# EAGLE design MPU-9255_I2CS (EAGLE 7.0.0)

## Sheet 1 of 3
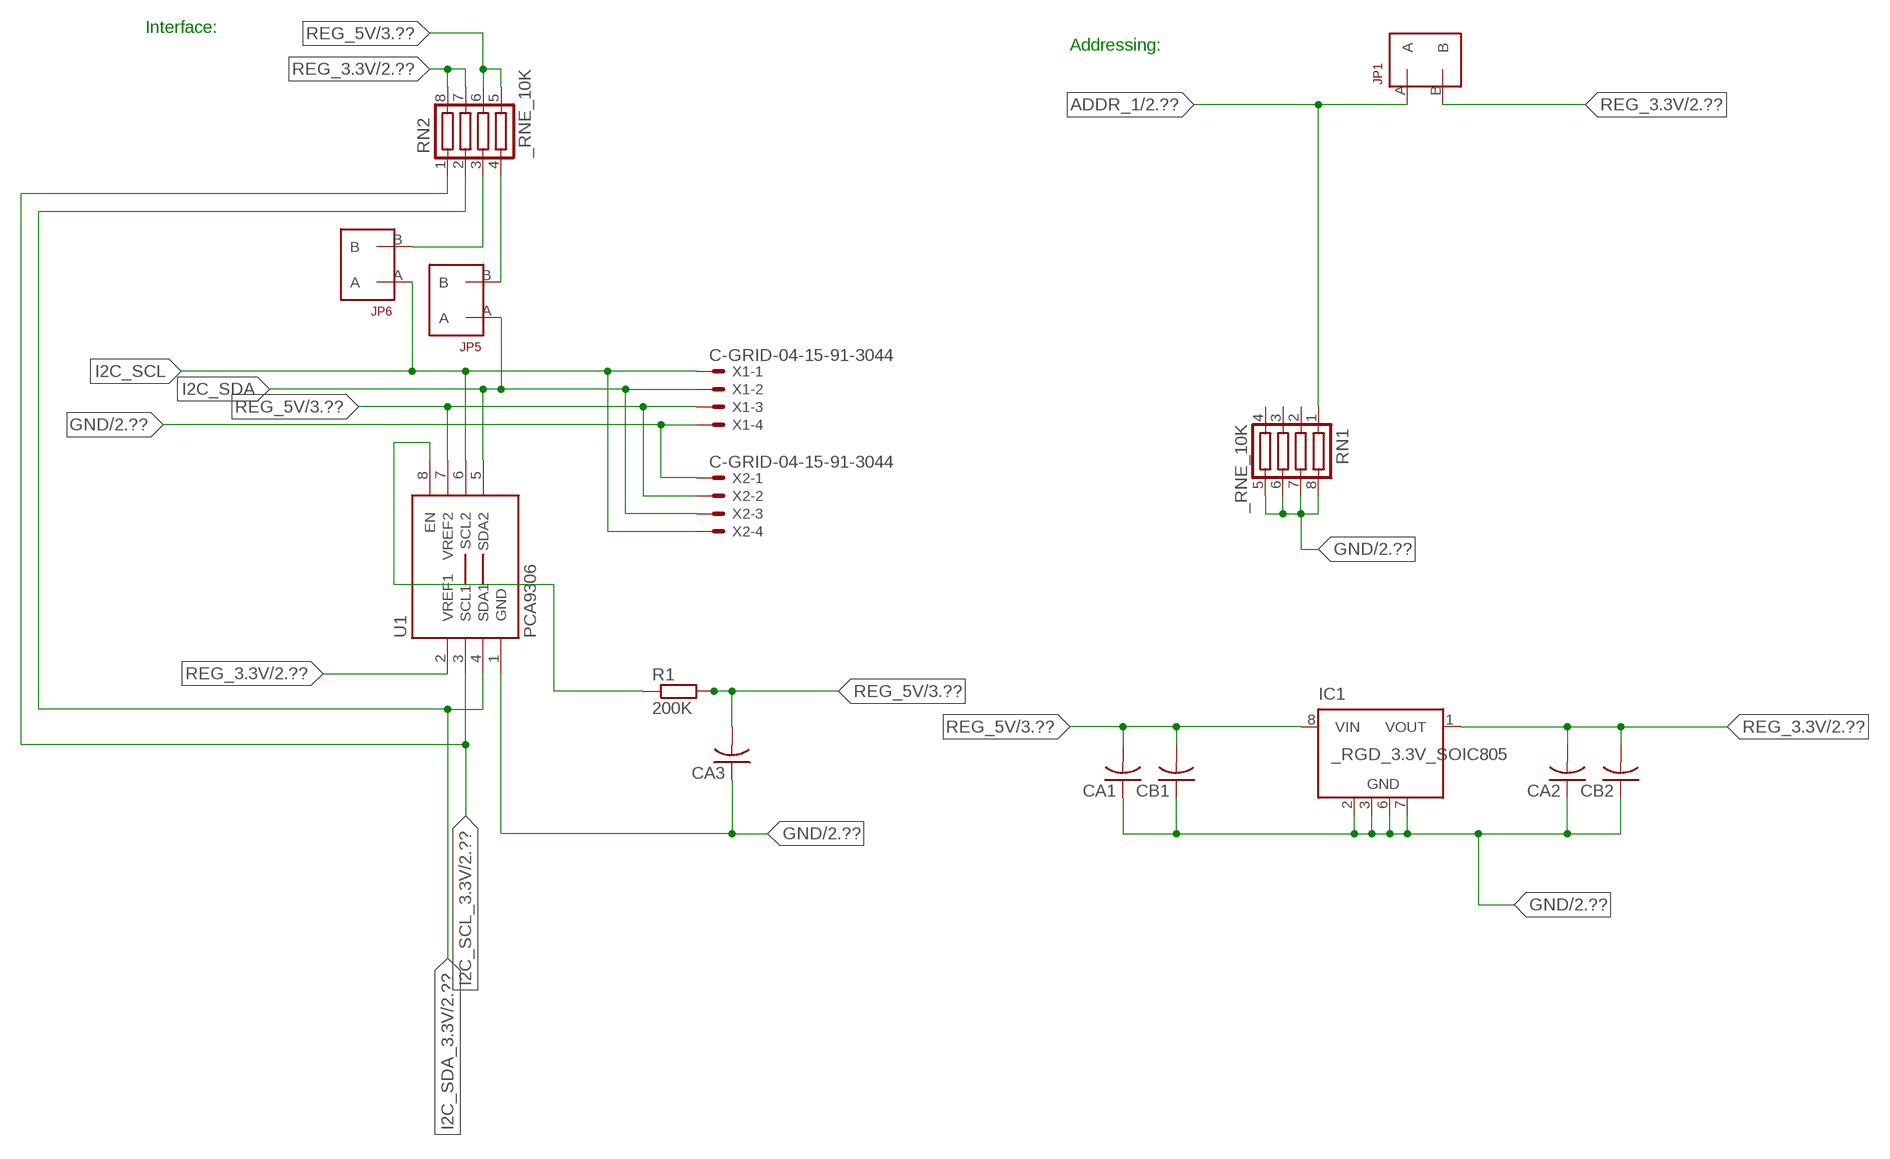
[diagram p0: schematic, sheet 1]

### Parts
CA1  CC1206KRX7R9BB104  [.1UF]
CA2  CC1206KRX7R9BB104  [.1UF]
CA3  CC1206KRX7R9BB104  [.1UF]
CB1  TMK316F106ZL-TC1206K  [TMK316F106ZL-T]
CB2  TMK316F106ZL-TC1206K  [TMK316F106ZL-T]
IC1  _RGD_3.3V_SOIC805  [_RGC_3.3V_SOIC8]
JP1  JUMPER_1X2_2MM  [JUMPER_1X2_2MM]
JP5  JUMPER_1X2_2MM  [JUMPER_1X2_2MM]
JP6  JUMPER_1X2_2MM  [JUMPER_1X2_2MM]
R1  200K  RESISTOR_SMT-0603  [R603]
RN1  _RNE_10K  [RNE]
RN2  _RNE_10K  [RNE]
U1  PCA9306  PCA9306_NCD  [PSOP-8]
X1  C-GRID-04-15-91-3044  [15-91-04]
X2  C-GRID-04-15-91-3044  [15-91-04]

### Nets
ADDR_1: JP1.A RN1.1 ; also sheet 2
GND: CA1.1 CA2.1 CA3.1 CB1.1 CB2.1 IC1.2(GND) IC1.3(GND) IC1.6(GND) IC1.7(GND) RN1.5 RN1.6 RN1.7 RN1.8 U1.1(GND) X1.4 X2.1 ; also sheet 2,3
I2C_SCL: JP6.A U1.6(SCL2) X1.1 X2.4
I2C_SCL_3.3V: RN2.1 U1.3(SCL1) ; also sheet 2
I2C_SDA: JP5.A U1.5(SDA2) X1.2 X2.3
I2C_SDA_3.3V: RN2.2 U1.4(SDA1) ; also sheet 2
N$1: JP6.B RN2.3
N$2: JP5.B RN2.4
N$3: R1.1 U1.8(EN)
REG_3.3V: CA2.2 CB2.2 IC1.1(VOUT) JP1.B RN2.7 RN2.8 U1.2(VREF1) ; also sheet 2
REG_5V: CA1.2 CA3.2 CB1.2 IC1.8(VIN) R1.2 RN2.5 RN2.6 U1.7(VREF2) X1.3 X2.2 ; also sheet 3
Unconnected: IC1.4(NC) IC1.5(NC) RN1.2 RN1.3 RN1.4

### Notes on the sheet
- Interface:
- Addressing:

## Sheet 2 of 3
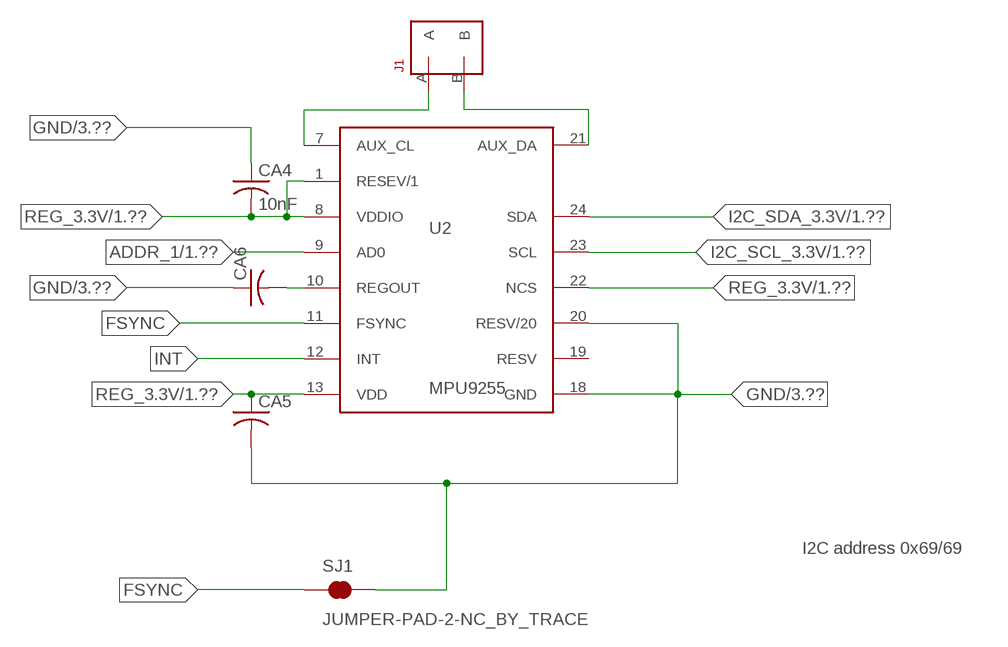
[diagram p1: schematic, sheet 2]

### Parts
CA4  10nF  CC1206KRX7R9BB104  [.1UF]
CA5  CC1206KRX7R9BB104  [.1UF]
CA6  CC1206KRX7R9BB104  [.1UF]
J1  JUMPER_1X2_2MM  [JUMPER_1X2_2MM]
SJ1  JUMPER-PAD-2-NC_BY_TRACE  [PAD-JUMPER-2-NC_BY_TRACE_YES_SILK]
U2  MPU9255  MPU_9255  [QFN-24]

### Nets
ADDR_1: U2.9(AD0) ; also sheet 1
FSYNC: SJ1.1 U2.11(FSYNC)
GND: CA4.1 CA5.2 CA6.1 SJ1.2 U2.18(GND) U2.20(RESV/20) ; also sheet 1,3
I2C_SCL_3.3V: U2.23(SCL) ; also sheet 1
I2C_SDA_3.3V: U2.24(SDA) ; also sheet 1
INT: U2.12(INT)
N$4: CA6.2 U2.10(REGOUT)
N$5: J1.A U2.7(AUX_CL)
N$6: J1.B U2.21(AUX_DA)
REG_3.3V: CA4.2 CA5.1 U2.1(RESEV/1) U2.8(VDDIO) U2.13(VDD) U2.22(NCS) ; also sheet 1
Unconnected: U2.19(RESV)

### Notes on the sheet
- I2C address 0x69/69

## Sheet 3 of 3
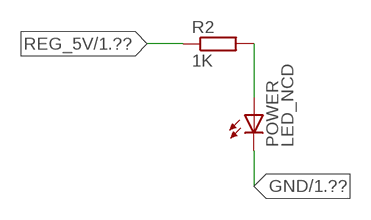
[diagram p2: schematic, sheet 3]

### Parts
POWER  LED_NCD  [CHIPLED_0603]
R2  1K  RESISTOR_SMT-0402  [R402]

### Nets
GND: POWER.C ; also sheet 1,2
N$7: POWER.A R2.2
REG_5V: R2.1 ; also sheet 1

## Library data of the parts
CA1-CA6 = NCD_ULTIMATE_LIBRARY:CC1206KRX7R9BB104: Capacitor CA .1uF 50V SMT C1206K CC1206KRX7R9BB104
CB1 CB2 = NCD_ULTIMATE_LIBRARY:TMK316F106ZL-T: Capacitor CB 10uF SMT 1206 TMK316F106ZL-T
IC1 = NCD_ULTIMATE_LIBRARY:_RGD_3.3V_SOIC8: Regulator Linear 3.3V Chip Positive VOLTAGE REGULATOR Digikey 497-1199-2-ND/L78L33ACD13TR
J1 JP1 JP5 JP6 = NCD_ULTIMATE_CONNECTORS:JUMPER_1X2_2MM
POWER = NCD_ULTIMATE_LIBRARY:LED_NCD: LED Digikey 754-1132-2-ND/APT2012SRCPRV
R1 R2 = NCD_ULTIMATE_LIBRARY:RESISTOR_SMT: NCD Resistor
RN1 RN2 = NCD_ULTIMATE_LIBRARY:_RNE_10K: Resistor Array RNE SMT 10K x 4 Single Resistor Source: http://www.ctscorp.com/components/Datasheets/CTSChipArrayDs.pdf Digikey 742C083103JPTR-ND/742C083103JP; OC_FARNELL: unknown; OC_NEWARK: unknown
SJ1 = NCD_ULTIMATE_CONNECTORS:JUMPER-PAD-2-NC_BY_TRACE
U1 = NCD_ULTIMATE_LIBRARY:PCA9306_NCD: NCD Bidirectional I2C level shifter. NOT compatible with all available part number pinout schemes- DOUBLE CHECK!!!; PROD_ID: IC-10023
U2 = NCD_ULTIMATE_bhaskar:MPU_9255: 9 Axis Sensor http://www.invensense.com/mems/gyro/documents/PS-MPU-9255.pdf
X1 X2 = NCD_ULTIMATE_CONNECTORS:C-GRID-04: CONNECTOR 4-Pos I2C wire to board 2.54 mm (0.100") pitch header Digikey WM1342-ND/0015912045; OC_FARNELL: unknown; OC_NEWARK: unknown

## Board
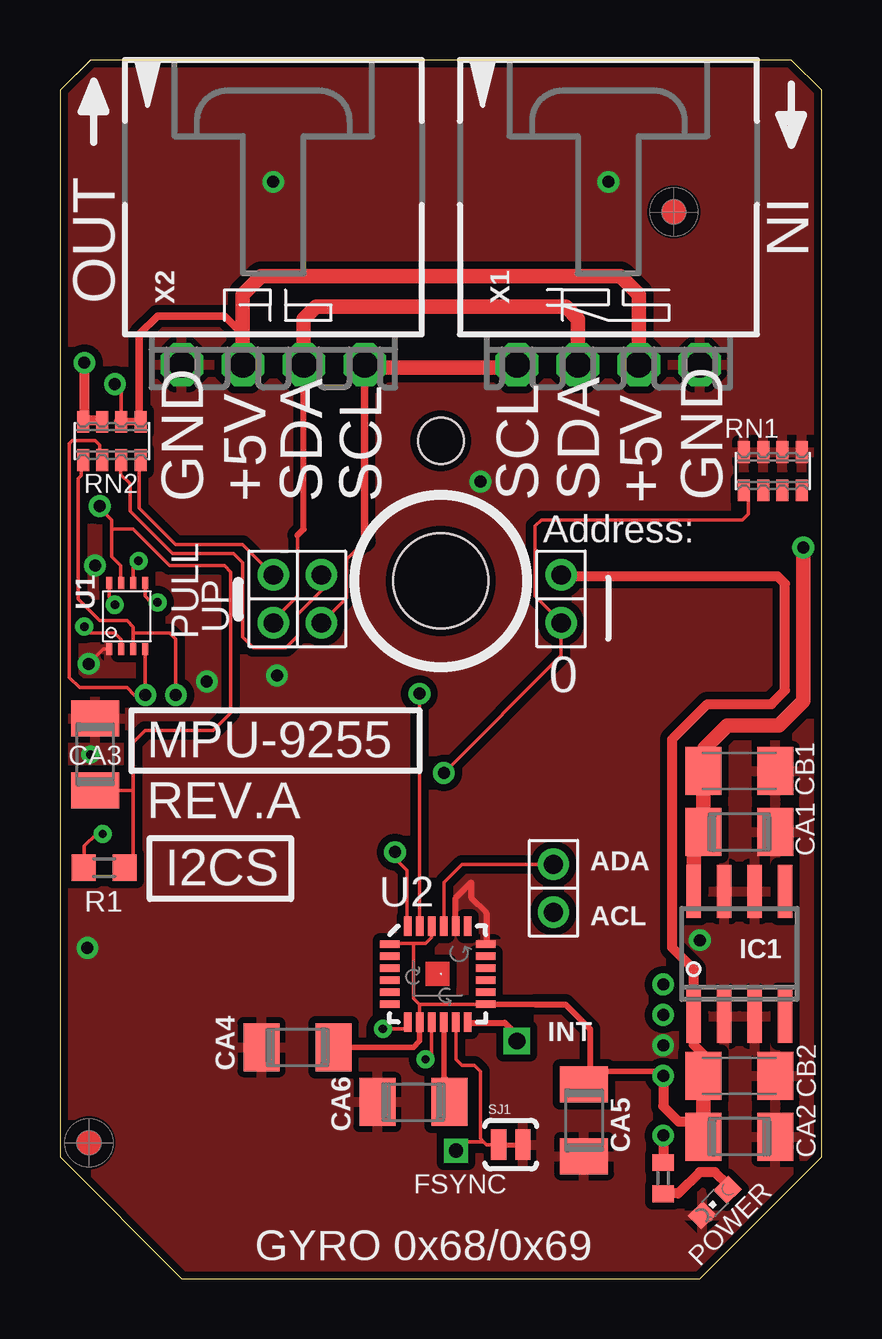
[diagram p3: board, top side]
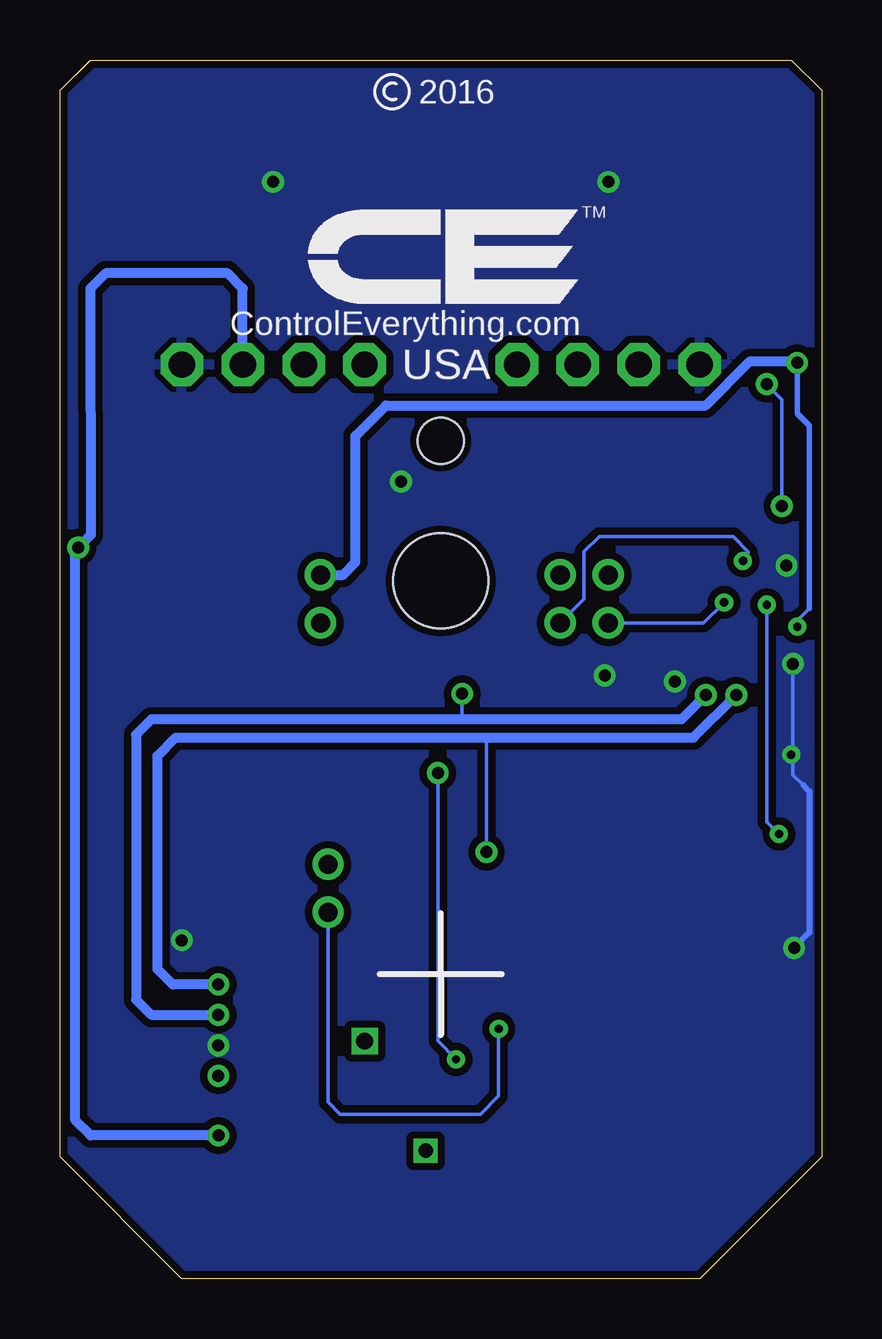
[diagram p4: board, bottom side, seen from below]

Size 31.75 x 50.8 mm. Coordinates in mm from the lower left corner, seen from the top.
Outline: 32 segments
Copper layers (1*16): Top 0.035mm / dielectric 1.5mm / Bottom 0.035mm
Design rules "default": minimum track width 5mil, minimum drill 24mil, track to track 5mil, track to pad 5mil, pad to pad 5mil, via to via 5mil, smd to smd 5mil, copper to edge 10mil, drill to drill 8mil, minimum pad ring 10mil, minimum via ring 8mil, stop-mask expansion 2mil, vias tented up to drill 0mil, thermal gap 10mil
Holes 3.96 mm at 15.88,29.08
Holes 1.91 mm at 15.88,34.93

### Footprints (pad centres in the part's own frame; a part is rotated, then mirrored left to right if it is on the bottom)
.1UF = smd 1.5 x 2: 1 -1.5,0; 2 1.5,0
TMK316F106ZL-T = smd 1.5 x 2: 1 -1.5,0; 2 1.5,0
_RGC_3.3V_SOIC8 = smd 0.6 x 2.2: 1 -1.905,-2.6; 2 -0.635,-2.6; 3 0.635,-2.6; 4 1.905,-2.6; 5 1.905,2.6; 6 0.635,2.6; 7 -0.635,2.6; 8 -1.905,2.6
JUMPER_1X2_2MM = drill 0.8: A 0,2; B 0,0
CHIPLED_0603 = smd 0.8 x 0.876: A 0,-0.75; C 0,0.75
R603 = smd 1 x 1.1: 1 -0.85,0; 2 0.85,0
R402 = smd 0.7 x 0.9: 1 -0.65,0; 2 0.65,0
RNE = smd 0.5 x 0.9: 1 -1.2,-0.8; 2 -0.4,-0.8; 3 0.4,-0.8; 4 1.2,-0.8; 5 1.2,0.8; 6 0.4,0.8; 7 -0.4,0.8; 8 -1.2,0.8
PAD-JUMPER-2-NC_BY_TRACE_YES_SILK = smd 0.635 x 1.27: 1 -0.508,0; 2 0.508,0
PSOP-8 = smd 0.25 x 0.5: 1 -0.73,-1.37; 2 -0.23,-1.37; 3 0.27,-1.37; 4 0.77,-1.37; 5 0.77,1.38; 6 0.27,1.38; 7 -0.23,1.38; 8 -0.73,1.38
QFN-24 = smd 0.8 x 0.3: 1 -2,1.25; 2 -2,0.75; 3 -2,0.25; 4 -2,-0.25; 5 -2,-0.75; 6 -2,-1.25; 13 2,-1.25; 14 2,-0.75; 15 2,-0.25; 16 2,0.25; 17 2,0.75; 18 2,1.25 | smd 0.3 x 0.8: 7 -1.25,-2; 8 -0.75,-2; 9 -0.25,-2; 10 0.25,-2; 11 0.75,-2; 12 1.25,-2; 19 1.25,2; 20 0.75,2; 21 0.25,2; 22 -0.25,2; 23 -0.75,2; 24 -1.25,2
15-91-04 = drill 1.1 pad 1.778 octagon: 1 -3.81,-7.62; 2 -1.27,-7.62; 3 1.27,-7.62; 4 3.81,-7.62

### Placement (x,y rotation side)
CA1  28.32,18.62 180 top
CA2  28.32,5.92 180 top
CA3  1.46,21.86 270 top
CA4  9.91,9.65 0 top
CA5  21.84,6.6 270 top
CA6  14.73,7.37 0 top
CB1  28.32,21.16 180 top
CB2  28.32,8.46 180 top
IC1  28.32,13.54 0 top
J1  20.57,17.27 180 top
JP1  20.89,29.34 180 top
JP5  8.89,29.34 180 top
JP6  10.9,29.34 180 top
POWER  27.3,3.18 135 top
R1  1.84,17.13 0 top
R2  25.15,4.19 270 top
RN1  29.72,33.66 0 top
RN2  2.16,34.93 0 top
SJ1  18.8,5.59 0 top
U1  2.79,27.61 0 top
U2  15.75,12.7 0 top
U$5  [VISION_REF10]  1.21,5.66 90 top
U$28  [VISION_REF10]  25.59,44.46 90 top
X1  22.86,45.72 0 top
X2  8.89,45.72 0 top

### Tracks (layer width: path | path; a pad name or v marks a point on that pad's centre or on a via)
ADDR_1  (via drill 0.35, 0.5)
  Top 0.152: RN1.1 28.7,32.78 28.7,31.88 28.45,31.62 20.07,31.62 19.81,31.37 19.81,28.45 20.89,27.37 JP1.A 20.89,25.97 v16,21.08 | U2.9 15.49,9.4 v15.24,9.14
  Bottom 0.152: v15.24,9.14 16,9.91 v16,21.08
FSYNC  (via drill 0.6)
  Top 0.152: U2.11 16.51,10.69 16.51,9.14 16.76,8.89 17.27,8.89 17.53,8.64 17.53,5.84 17.65,5.72 | 17.65,5.72 17.78,5.59 SJ1.1 | v16.51,5.33 16.89,5.72 17.65,5.72
GND  (via drill 0.35, 0.5)
  Top 0.152: CA3.1 1.52,23.42 1.52,23.62 | v1.19,25.63 1.8,26.24 U1.1
  Top 0.254: U2.20 16.5,15.86 17.14,16.51 17.14,15.88 17.78,15.24 17.78,13.98 U2.18
  Bottom 0.152: 0.76,20.57 1.19,21.01 v1.19,25.63
  Bottom 0.254: 0.76,20.57 0.51,20.32 0.51,14.43 v1.15,13.79
  other vias: 8.89,45.72 22.86,45.72 25.15,9.73 1.46,29.73 17.53,33.22 26.67,14.11 9.04,25.15 6.12,24.89 1.27,21.84
  pour Bottom (isolate 0.305): -0.64,5.08 -0.64,49.53 1.27,51.44 30.48,51.44 32.38,49.53 32.38,5.08 26.67,-0.63 5.08,-0.63
  pour Top (isolate 0.305): 4.45,-1.27 -1.27,4.45 -1.27,50.17 0.64,52.07 31.11,52.07 33.02,50.17 33.02,4.45 27.3,-1.27
I2C_SCL  (via drill 0.35)
  Top 0.152: 12.7,30.73 11.94,29.97 11.94,28.38 JP6.A | v3.28,29.92 3.06,29.96 U1.6
  Top 0.305: 12.7,30.73 X2.4
  Top 0.406: X2.4 12.7,37.97 | 19.05,37.97 X1.1
  Top 0.61: 12.7,37.97 19.05,37.97
  Bottom 0.152: JP6.A 9.91,28.33 9.91,30.3 9.27,30.94 3.69,30.94 3.05,30.3 v3.28,29.92
I2C_SCL_3.3V  (via drill 0.5)
  Top 0.152: RN2.1 0.89,34.07 0.89,33.48 0.77,33.35 0.77,28.33 1.67,27.43 2.79,27.43 3.06,27.17 3.06,26.92 | U2.23 14.99,14.71 v14.99,24.38 | 3.06,26.92 U1.3 | v4.83,24.33 v4.83,24.34 4.83,26.67 4.57,26.92 3.06,26.92
  Bottom 0.152: v14.99,24.38 14.99,23.32
  Bottom 0.406: v4.83,24.33 5.84,23.32 14.99,23.32 27.94,23.32 28.58,22.68 28.58,11.63 27.94,11 v25.15,11
I2C_SDA  (via drill 0.35)
  Top 0.152: JP5.A 8.89,27.44 9.91,28.45 9.91,30.99 | U1.5 3.56,28.45 3.81,28.19 v4.06,28.19
  Top 0.254: 9.91,30.99 10.16,31.25 X2.3
  Top 0.61: X2.3 10.16,40.01 10.67,40.51 21.09,40.51 21.59,40.01 X1.2
  Bottom 0.152: v4.06,28.19 4.92,27.34 JP5.A
I2C_SDA_3.3V  (via drill 0.5)
  Top 0.152: RN2.2 1.65,34.14 1.65,34.75 1.46,34.94 0.51,34.94 0.38,34.81 0.38,26.37 0.38,26.36 0.38,25.07 0.81,24.64 2.79,24.64 3.1,24.33 v3.56,24.33 v3.56,24.34 U1.4 | U2.24 14.48,14.72 14.48,17.02 13.97,17.53 v13.97,17.78
  Bottom 0.152: v13.97,17.78 13.97,22.56
  Bottom 0.406: v25.15,12.27 27.05,12.27 27.69,12.9 27.69,21.79 26.93,22.56 13.97,22.56 5.34,22.56 v3.56,24.33
INT  (via drill 0.7)
  Top 0.254: U2.12 17.03,10.67 18.54,10.67 19.05,10.16 v19.05,9.91
N$1
  Top 0.152: JP6.B 10.92,29.31 10.92,28.7 9.91,27.69 9.91,26.8 9.42,26.31 8.06,26.31 7.62,26.75 7.62,29.84 7.24,30.23 4.7,30.23 2.92,32 2.92,33.15 2.54,33.53 2.54,34.1 RN2.3
  Top 0.305: 2.54,34.02 RN2.3
N$2
  Top 0.152: JP5.B 7.62,30.61 4.83,30.61 3.3,32.13 3.3,34.07 RN2.4
  Top 0.305: 3.37,33.88 RN2.4
N$3  (via drill 0.35)
  Top 0.152: R1.1 1.02,17.16 1.02,18.03 1.52,18.54 v1.78,18.54 | v2.29,28.09 2.06,28.42 U1.8
  Bottom 0.152: v1.78,18.54 2.29,19.05 v2.29,28.09
N$4
  Top 0.229: U2.10 16,8.38 16.23,8.15 CA6.2
N$5  (via drill 0.35)
  Top 0.152: U2.7 14.48,10.68 14.48,10.41 v13.46,10.41
  Bottom 0.152: v13.46,10.41 13.46,7.62 14.22,6.86 20.07,6.86 20.57,7.37 J1.A
N$6
  Top 0.152: U2.21 16,16.51 16.76,17.27 J1.B
N$7
  Top 0.406: POWER.A 27.84,3.92 27.3,4.45 26.67,4.45 25.78,3.56 25.16,3.56 R2.2
REG_3.3V  (via drill 0.35, 0.5)
  Top 0.152: U2.1 13.77,13.97 14.73,13.97 | 14.73,13.97 15.24,13.97 15.5,14.23 U2.22 | U2.8 14.99,10.71 14.99,11.43 | 14.99,11.43 14.73,11.68 14.73,13.97 | U2.13 17.73,11.43 14.99,11.43 | v1.02,27.18 1.27,26.92 2.29,26.92 2.56,26.65 U1.2
  Top 0.229: U2.13 17.77,11.43 19.81,11.43 | v25.15,8.46 24.97,8.64 22.1,8.64 22.1,7.87 22.12,7.85 CA5.1 | CA4.2 14.73,9.65 15,9.92 U2.8
  Top 0.254: 19.81,11.43 21.08,11.43 22.1,10.41 22.1,8.64
  Top 0.406: CB2.2 26.82,9.35 26.42,9.75 26.42,10.36 | v25.15,8.46 25.15,7.19 25.78,6.55 26.82,6.55 | IC1.1 26.42,12.9 25.53,13.79 25.53,22.49 26.99,23.95 29.66,23.95 30.23,24.52 30.23,28.97 29.91,29.29 20.95,29.29 JP1.B | 26.52,5.62 CA2.2 | v1.02,38.18 1.02,35.78 | 1.02,35.78 RN2.8 | 1.02,35.78 1.71,35.78 RN2.7
  Top 0.61: CB2.2 26.82,6.55 CA2.2 | 26.42,10.36 IC1.1
  Bottom 0.152: 0.51,27.94 1.02,27.43 v1.02,27.18
  Bottom 0.229: 0.51,27.94 0.51,35.56 1.02,36.07 v1.02,38.18
  Bottom 0.406: v1.02,38.18 1.08,38.24 2.99,38.24 4.83,36.4 18.16,36.4 19.43,35.13 19.43,29.87 19.94,29.34 JP1.B
REG_5V  (via drill 0.5)
  Top 0.152: RN2.6 2.56,37.01 v2.29,37.29 | R1.2 3.05,17.49 3.05,20.36 | 3.05,20.36 3.05,22.35 3.56,22.86 6.39,22.86 7.11,23.58 7.11,29.46 6.86,29.72 4.57,29.72 3.05,31.24 2.16,31.24 | CA3.2 3.05,20.36 | v1.65,32.21 1.65,32.13 2.16,31.62 2.16,31.24 | U1.7 2.54,29.01 2.54,29.72 2.16,30.1 2.16,31.24
  Top 0.305: 7.62,39.37 7.5,39.37 | 2.42,35.74 RN2.6 RN2.5 3.31,35.8 3.31,39.37 4.07,40.13 6.86,40.13 7.62,39.37 | X2.2 7.62,39.37
  Top 0.406: v25.15,5.97 R2.1 | 24.13,38.23 X1.3
  Top 0.61: X2.2 7.62,41.02 8.38,41.78 23.37,41.78 24.13,41.02 24.13,38.23 | IC1.8 26.42,18.21 CA1.2 CB1.2 26.86,21.2 26.86,22.11 27.82,23.06 29.98,23.06 30.99,24.08 v30.99,30.48
  Bottom 0.152: v1.65,32.21 1.65,36.65 v2.29,37.29
  Bottom 0.406: X1.3 24.13,41.28 24.77,41.91 29.84,41.91 30.48,41.27 30.47,31 v30.99,30.48 31.11,30.36 31.11,6.6 30.48,5.97 v25.15,5.97

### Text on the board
tNames: IN | OUT | GND | +5V | SDA | SCL | SCL | SDA | +5V | GND | Address: | PULL | UP | 0 | MPU-9255 | REV.A | ADA | I2CS | ACL | INT | FSYNC | GYRO 0x68/0x69
bNames: 2016 | TM | ControlEverything.com | USA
